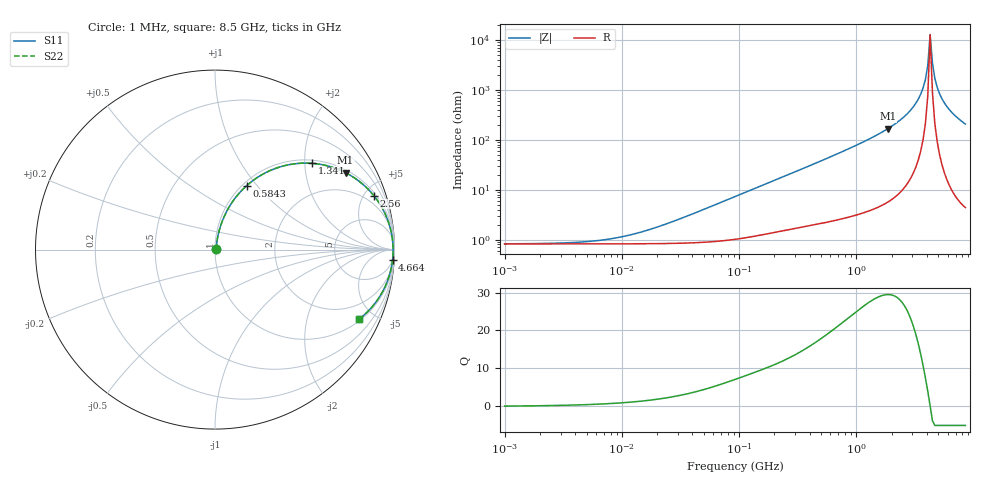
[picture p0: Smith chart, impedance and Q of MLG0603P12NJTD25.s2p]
! S-Parameter Data Generated by TDK Corporation
! Copyright(C) 2025 TDK Corporation.
! All Rights Reserved.
! TDK P/N: MLG0603P12NJTD25 (SMD / SMT Inductor (Coil))
! Property: L=12nH at 500MHz
! Size(LxWxT): 0.6x0.3x0.3mm
! Model Type: s2p (Touchstone File Format Version 1.0)
! Frequency: DC=Yes Start=1MHz Stop=8500MHz 198points Log-sweep
! Model Generated on Feb. 6, 2025
! Terms and conditions regarding TDK Simulation Models:
! 1)This simulation model is being provided solely for informational
!  purposes. Please refer to the specifications of the products in
!  terms of detailed characteristics of such products.
! 2)In no event shall TDK Corporation of any of its subsidiaries be
!  liable for any loss or damage arising, directly or indirectly,
!  from any information contained in this simulation model, including,
!  but not limited to loss or damages arising from any inaccuracies,
!  omissions or errors in connection with such information.
! 3)Any and all copyrights on this simulation model are owned by
!  TDK Corporation.  Duplication or redistribution of this simulation
!  model without prior written permission from TDK Corporation
!  is prohibited.
! 4)This simulation model is subject to any modification or change
!  without any prior notice.
! 5)Neither TDK Corporation nor any of its subsidiaries shall make any
!  warranty, express or implied, including but not limited to the
!  correctness, implied warranties of merchantability and fitness for
!  a particular purpose with respect to this simulation models.
! 6)The use of this simulation model shall be deemed to have consented
!  to the terms and conditions hereof.
! Port Assignments:
!  1 ---@@@--- 2
! Applicable Conditions:
!  Temperature = 25 degC
!  DC Bias Current = 0 A
!  Small Signal Operation
# Hz S MA R 50
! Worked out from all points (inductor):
!   197 points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, 1 MHz to 8.5 GHz, reference 50 ohm
!   read as one part in series: L = 12.5 nH near 33.39 MHz
!   highest Q = 29.4 at 1.853 GHz (marker M1), where L = 14.3 nH
!   self-resonance near 4.253 GHz
!   S11 on the Smith chart (normalised r, x): 1 MHz: 1.02, +0.00; 584.3 MHz: 1.05, +0.88; 1.341 GHz: 1.08, +2.18; 2.56 GHz: 1.22, +5.81; 4.664 GHz: 5, -34; 8.5 GHz: 1.09, -4.12
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1000000  0.008171 5.5  0.9919 -0.0  0.9919 -0.0  0.008171 5.5
4587603  0.008897 23.6  0.9919 -0.2  0.9919 -0.2  0.008897 23.6
1.005548e7  0.01134 43.5  0.9918 -0.5  0.9918 -0.5  0.01134 43.5
2.10461e7  0.01842 62.4  0.9916 -0.9  0.9916 -0.9  0.01842 62.4
9.219544e7  0.07179 77.9  0.9875 -4.1  0.9875 -4.1  0.07179 77.9
4.229561e8  0.2991 69.1  0.9361 -17.4  0.9361 -17.4  0.2991 69.1
5.842944e8  0.3967 63.7  0.8977 -23.3  0.8977 -23.3  0.3967 63.7
1.34121e9  0.7236 41.6  0.6648 -46.3  0.6648 -46.3  0.7236 41.6
1.852819e9  0.8445 30.5  0.5076 -57.6  0.5076 -57.6  0.8445 30.5
1.940355e9  0.8597 28.8  0.4825 -59.2  0.4825 -59.2  0.8597 28.8
2.559585e9  0.9348 18.8  0.3217 -69.1  0.3217 -69.1  0.9348 18.8
3.224109e9  0.9745 10.3  0.1786 -76.7  0.1786 -76.7  0.9745 10.3
3.703002e9  0.9875 5.2  0.09068 -79.5  0.09068 -79.5  0.9875 5.2
3.877948e9  0.9901 3.5  0.06127 -78.9  0.06127 -78.9  0.9901 3.5
4.061159e9  0.9917 1.8  0.03207 -74.1  0.03207 -74.1  0.9917 1.8
4.253027e9  0.9924 0.1  0.007735 -10.5  0.007735 -10.5  0.9924 0.1
4.453958e9  0.9922 -1.6  0.02924 73.7  0.02924 73.7  0.9922 -1.6
4.664383e9  0.991 -3.3  0.05845 79.5  0.05845 79.5  0.991 -3.3
5.115526e9  0.986 -6.7  0.1176 79.8  0.1176 79.8  0.986 -6.7
5.610304e9  0.9772 -10.2  0.1766 77.5  0.1766 77.5  0.9772 -10.2
6.748056e9  0.9485 -17.0  0.2931 71.5  0.2931 71.5  0.9485 -17.0
8.5e9  0.8923 -25.6  0.4328 63.1  0.4328 63.1  0.8923 -25.6
